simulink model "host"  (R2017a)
settings: Solver=FixedStepDiscrete  StartTime=0.0  StopTime=1000  FixedStep=0.01  RelTol=1e-3  EnableMultiTasking=on
undefined symbols (not defined in the file): COM
libraries: c2000scilib x3

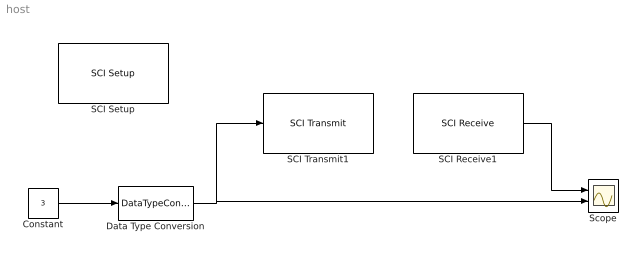
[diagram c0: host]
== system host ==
  Constant : Constant  Value=3
  Data Type Conversion : DataTypeConversion  OutDataTypeStr=single
  SCI Receive1 : c2000scilib/SCI Receive  module=COM 2  dataHead='S'  dataTail='E'  dataType=single  dataDim=1  initValue=0  errOption=Output the last received value  errValue=0  sampleTime=-1  outputStatus=off
  SCI Setup : c2000scilib/SCI Setup  Priority=-99  commModeA=raw data  baudRateA=115200  charLenA=8  stopBitA=1  parityA=none  timeoutA=1.0  commModeB=raw data  baudRateB=115200  charLenB=8  stopBitB=1  parityB=none  timeoutB=1.0  commModeC=raw data  baudRateC=115200  charLenC=8  stopBitC=1  parityC=none  timeoutC=1.0  commModeD=raw data  baudRateD=115200  charLenD=8  stopBitD=1  parityD=none  timeoutD=1.0
  SCI Transmit1 : c2000scilib/SCI Transmit  module=COM 2  header='S'  tail='E'
  Scope : Scope  NumInputPorts=2
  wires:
  Data Type Conversion/1 -> SCI Transmit1/1, Scope/2
  SCI Receive1/1 -> Scope/1
  Constant/1 -> Data Type Conversion/1
